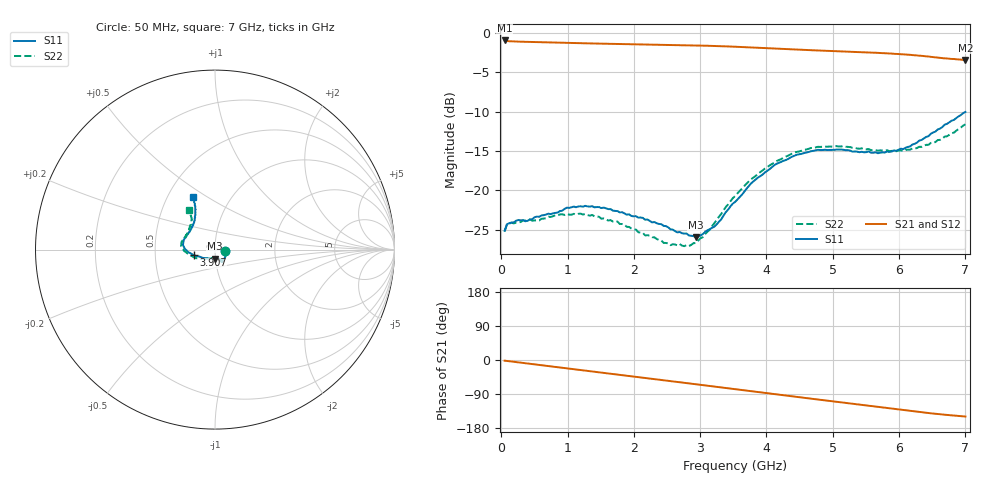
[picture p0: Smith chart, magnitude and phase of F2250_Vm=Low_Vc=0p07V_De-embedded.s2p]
! Integrated Device Technology
! Corporate Headquarters
! 6024 Silver Creek Valley Road
! San Jose, CA 95138  USA
! Phone:  1-408-284-8200
! Toll Free:  1-800-223-1366
! Webpage:  http://www.idt.com/
! Timing and RF Division
! 515 Groton Road, Suite 102
! Westford, MA 01886-6024
! Device:  F2250
! Description: Voltage Variable RF Attenuator
! Frequency:  50.0 -  6000.00 MHz
! Package:  3x3 mm Thin QFN Plastic Package: 16 pin
! Ports:  2 RF, 3 DC
!  Pin  1  = GND
!  Pin  2  = NC
!  Pin  3  = RF1  = Port 1
!  Pin  4  = NC
!  Pin  5  = GND
!  Pin  6  = GND
!  Pin  7  = GND
!  Pin  8  = GND
!  Pin  9  = NC
!  Pin 10  = RF2  = Port 2
!  Pin 11  = NC
!  Pin 12  = GND
!  Pin 13  = GND
!  Pin 14  = VCNTRL
!  Pin 15  = VDD
!  Pin 16  = VMODE
! Vcntrl:  0.070 Volts
! Vmode:  +0.000 Volts
! Vdd:  +3.30  Volts
! Current:  1.106 mA
! Data:  The device was measured on a the F2250 evaluation board which has
!  individual transmission lines to the RF pins.  Data was collected
!  using a calibrated network analyzer.  The evaluation board was
!  de-embedded using a TRL calibration technique.
!  The reference plane is the edge of the package pin.
! Misc:  SN 10
!  Action Tracker AT0258
! Date Measured:  2014-11-26
! Date:  2015-10-15  MJV
! Note:
!  Integrated Device Technology supplies this data as a sample of measured
!  data at the package pin for this product.  Your particular data for this
!  product may vary.
!  Data was taken at 25 degrees C.
!  Integrated Device Technology reserves the right to change this data at anytime.
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# GHz S dB R 50
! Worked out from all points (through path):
!   201 points, 50 MHz to 7 GHz, reference 50 ohm
!   highest |S21| = -0.93 dB at 50 MHz (marker M1); lowest = -3.4 dB at 7 GHz (marker M2)
!   group delay of S21, straight-line fit = 59.9 ps
!   lowest |S11| = -26.0 dB at 2.934 GHz (marker M3), VSWR 1.11, Z = 49.5 - j5 ohm
!   |S11| at or under -10 dB: start of sweep to end of sweep
!   |S22| runs from -27.1 to -11.6 dB; largest |S21 - S12| = 0.00033
!   S11 on the Smith chart (normalised r, x): 50 MHz: 1.12, -0.02; 3.907 GHz: 0.79, -0.05; 7 GHz: 0.67, +0.43
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0.05  -25.12 -9.7  -0.93 -1.8  -0.93 -1.8  -25.23 -10.1
0.08475  -24.29 -9.7  -0.99 -2.5  -0.99 -2.5  -24.35 -9.4
0.15425  -24.07 -11.9  -1.04 -4.0  -1.04 -3.9  -24.11 -11.0
0.57125  -23.35 -30.1  -1.14 -13.1  -1.14 -13.1  -23.82 -30.4
0.884  -22.62 -45.9  -1.20 -19.9  -1.20 -19.9  -23.05 -46.8
1.2315  -22.06 -56.1  -1.28 -27.4  -1.28 -27.3  -23.06 -59.7
1.75275  -22.62 -62.8  -1.37 -38.4  -1.37 -38.4  -23.95 -66.7
2.37825  -24.26 -63.6  -1.46 -51.8  -1.46 -51.8  -26.29 -67.8
2.552  -24.94 -67.8  -1.49 -55.6  -1.49 -55.6  -26.95 -73.3
2.83  -25.72 -83.3  -1.54 -61.7  -1.54 -61.7  -27.07 -92.6
2.93425  -25.96 -92.4  -1.56 -64.0  -1.56 -64.0  -26.69 -101.5
3.21225  -24.62 -122.1  -1.63 -70.1  -1.63 -70.1  -24.17 -127.6
3.525  -21.47 -148.3  -1.72 -77.0  -1.72 -77.0  -20.72 -146.4
3.76825  -19.10 -161.3  -1.81 -82.4  -1.81 -82.4  -18.56 -156.7
3.90725  -18.17 -165.6  -1.87 -85.4  -1.87 -85.4  -17.66 -162.8
4.1505  -16.61 -173.7  -1.97 -90.7  -1.96 -90.7  -16.27 -171.4
4.7065  -14.96 172.3  -2.18 -102.7  -2.18 -102.7  -14.60 175.7
5.15825  -14.82 161.5  -2.33 -112.5  -2.33 -112.5  -14.37 166.6
5.85325  -15.10 138.4  -2.58 -127.4  -2.58 -127.4  -15.00 151.6
6.166  -14.40 127.6  -2.75 -134.2  -2.75 -134.2  -14.81 142.7
6.444  -13.10 119.3  -2.96 -140.0  -2.96 -140.0  -14.19 133.4
7  -10.01 113.1  -3.41 -149.2  -3.41 -149.2  -11.59 123.9
